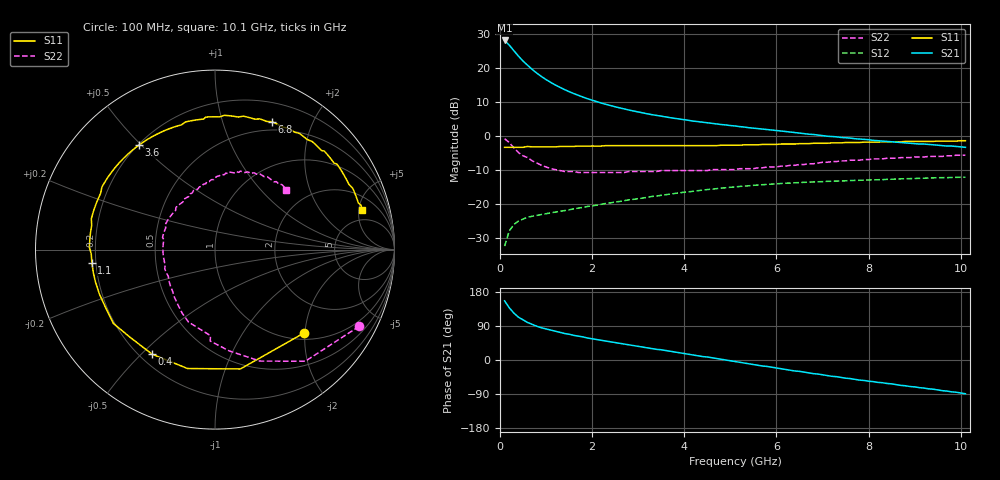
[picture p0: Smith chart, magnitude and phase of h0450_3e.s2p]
!HBFP-0450
!S and NOISE PARAMETERS at Vce=3V  Ic=15mA.  LAST UPDATED  09-04-98
# GHZ S MA R  50
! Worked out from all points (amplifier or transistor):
!   101 points, 100 MHz to 10.1 GHz, reference 50 ohm
!   highest |S21| = 28.0 dB at 100 MHz (marker M1)
!   |S21| within 3 dB of that: start of sweep to 300.5 MHz
!   unconditionally stable (mu >= 1): 2.584 GHz to end of sweep
!   at 1.7 GHz: K = 0.83, MSG = 16.6 dB, |S12| = -21.2 dB
!   at 5.1 GHz: K = 1.13, MAG = 6.7 dB, |S12| = -15.0 dB
!   at 10.1 GHz: K = 1.07, MAG = 2.8 dB, |S12| = -12.1 dB
!   lowest NFmin = 1.17 dB at 1.8 GHz
!   S11 on the Smith chart (normalised r, x): 100 MHz: 1.15, -1.98; 400 MHz: 0.25, -0.54; 1.1 GHz: 0.18, -0.05; 3.6 GHz: 0.20, +0.49; 6.8 GHz: 0.40, +1.46; 10.1 GHz: 3.45, +5.47
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0.1  0.68 -43.0  25.26 156.0  0.024 69.0  0.91 -28.0
0.2  0.68 -78.0  21.6 138.0  0.04 54.0  0.8 -51.0
0.3  0.68 -103.0  17.9 124.0  0.05 46.0  0.67 -68.0
0.4  0.68 -121.0  14.89 113.0  0.056 39.0  0.57 -82.0
0.5  0.68 -134.0  12.57 106.0  0.06 35.0  0.51 -93.0
0.6  0.7 -144.0  10.9 99.0  0.064 32.0  0.48 -93.0
0.7  0.69 -152.0  9.47 94.0  0.066 31.0  0.43 -110.0
0.8  0.69 -159.0  8.35 89.0  0.068 30.0  0.4 -117.0
0.9  0.69 -165.0  7.45 85.0  0.07 29.0  0.37 -124.0
1.1  0.69 -174.0  6.12 79.0  0.074 29.0  0.33 -136.0
1.4  0.7 175.0  4.8 70.0  0.08 28.0  0.3 -150.0
1.6  0.7 169.0  4.19 65.0  0.085 28.0  0.3 -159.0
1.8  0.71 163.0  3.72 61.0  0.089 28.0  0.29 -166.0
2.1  0.71 156.0  3.19 54.0  0.096 27.0  0.29 -176.0
2.5  0.72 147.0  2.68 46.0  0.107 25.0  0.29 174.0
3  0.72 137.0  2.25 36.0  0.12 22.0  0.3 163.0
3.5  0.72 128.0  1.95 27.0  0.134 19.0  0.31 154.0
3.6  0.72 126.0  1.9 25.0  0.137 18.0  0.31 152.0
5.1  0.73 97.0  1.4 -4.0  0.178 1.0  0.32 124.0
6.8  0.78 66.0  1.05 -36.0  0.211 -22.0  0.39 91.0
8.5  0.82 39.0  0.82 -63.0  0.231 -44.0  0.47 66.0
10.1  0.85 15.0  0.68 -89.0  0.247 -66.0  0.52 40.0
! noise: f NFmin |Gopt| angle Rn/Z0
1.8  1.17  0.48  -171  0.05
2  1.22  0.5  -167  0.05
2.5  1.36  0.53  -154  0.08
3.5  1.65  0.6  -134  0.17
4  1.83  0.62  -122  0.27
5  2.14  0.66  -101  0.57
5.5  2.29  0.7  -90  0.8
7  2.73  0.75  -61  1.81
8  3.08  0.79  -44  2.74
10  3.63  0.81  -15  4.59
